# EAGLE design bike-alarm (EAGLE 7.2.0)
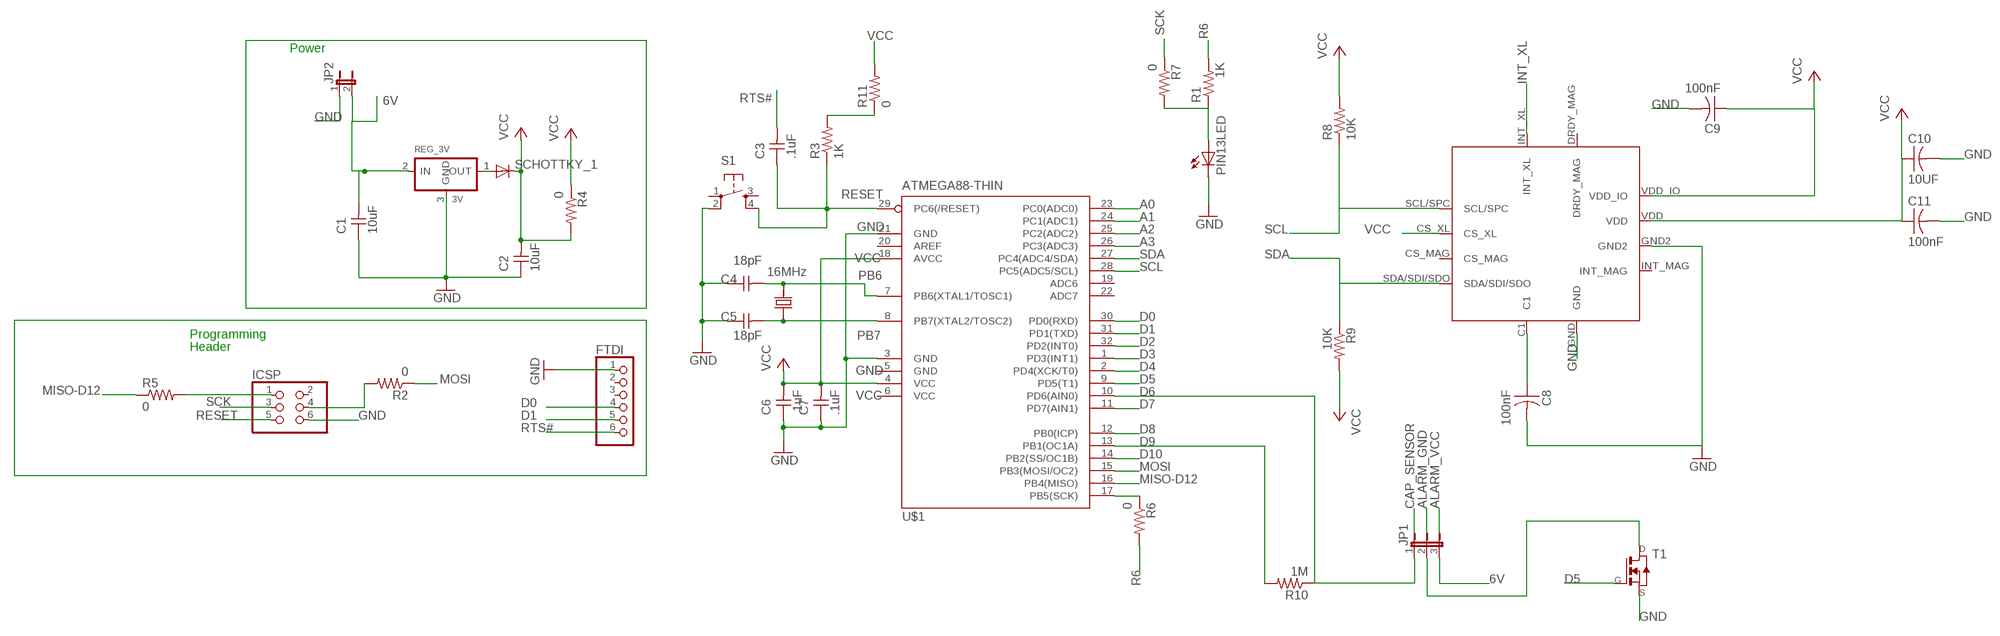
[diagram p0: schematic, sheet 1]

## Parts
C1  10uF  UNPOLARIZED_CAPACITOR1206  [1206]
C2  10uF  UNPOLARIZED_CAPACITOR1206  [1206]
C3  .1uF  UNPOLARIZED_CAPACITOR1206  [1206]
C4  18pF  UNPOLARIZED_CAPACITOR1206  [1206]
C5  18pF  UNPOLARIZED_CAPACITOR1206  [1206]
C6  .1uF  UNPOLARIZED_CAPACITOR1206  [1206]
C7  .1uF  UNPOLARIZED_CAPACITOR1206  [1206]
C8  100nF  CAP-US1206FAB  [C1206FAB]
C9  100nF  CAP-US1206FAB  [C1206FAB]
C10  10UF  CAP-US1206FAB  [C1206FAB]
C11  100nF  CAP-US1206FAB  [C1206FAB]
FTDI  PINHD-1X6  [1X06]
ICSP  PINHD-2X3-SMD  [2X03SMD]
JP1  JP2E  [JP2]
JP2  JP1E  [JP1]
PIN13LED  LED1206  [1206]
Q2  16MHz  CRYSTALCS10  [CS10]
R1  1K  RESISTOR1206  [1206]
R2  0  RES-US1206FAB  [R1206FAB]
R3  1K  RESISTOR1206  [1206]
R4  0  RES-US1206FAB  [R1206FAB]
R5  0  RES-US1206FAB  [R1206FAB]
R6  0  RES-US1206FAB  [R1206FAB]
R7  0  RES-US1206FAB  [R1206FAB]
R8  10K  RES-US1206FAB  [R1206FAB]
R9  10K  RES-US1206FAB  [R1206FAB]
R10  1M  RES-US1206FAB  [R1206FAB]
R11  0  RES-US1206FAB  [R1206FAB]
REG_3V  3V  REGULATORSOT23  [SOT23]
S1  6MM_SWITCH6MM_SWITCH  [6MM_SWITCH]
SCHOTTKY_1  DIODESOD123  [SOD123]
T1  NMOSFETSOT23  [SOT-23]
U$1  ATMEGA88-THIN  [TQFP32-08THIN]
U$3  LSM303C  [LSM303C]

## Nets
6V: C1.2 JP1.3 JP2.2 REG_3V.2(IN)
A: JP1.2 T1.1(D)
A0: U$1.23(PC0(ADC0))
A1: U$1.24(PC1(ADC1))
A2: U$1.25(PC2(ADC2))
A3: U$1.26(PC3(ADC3))
D0: FTDI.4 U$1.30(PD0(RXD))
D1: FTDI.5 U$1.31(PD1(TXD))
D2: U$1.32(PD2(INT0))
D3: U$1.1(PD3(INT1))
D4: U$1.2(PD4(XCK/T0))
D5: T1.3(G) U$1.9(PD5(T1))
D6: JP1.1 R10.1 U$1.10(PD6(AIN0))
D7: U$1.11(PD7(AIN1))
D8: U$1.12(PB0(ICP))
D9: R10.2 U$1.13(PB1(OC1A))
D10: U$1.14(PB2(SS/OC1B))
GND [power]: C1.1 C2.1 C4.1 C5.1 C6.1 C7.1 C8.2 C9.2 C10.2 C11.2 FTDI.1 ICSP.6 JP2.1 PIN13LED.2(C) REG_3V.3(GND) S1.2(P1) T1.2(S) U$1.3(GND) U$1.21(GND) U$3.GND U$3.GND2
INT_XL: U$3.INT_XL
MISO-D12: R5.1 U$1.16(PB4(MISO))
MOSI: R2.1 U$1.15(PB3(MOSI/OC2))
N$1 [power]: REG_3V.1(OUT) SCHOTTKY_1.ANODE(A)
N$4: PIN13LED.1(A) R1.1 R7.2
N$6: C8.1 U$3.C1
N$8: ICSP.4 R2.2
N$21: ICSP.1 R5.2
PB6: C4.2 Q2.P$2 U$1.7(PB6(XTAL1/TOSC1))
PB7: C5.2 Q2.P$1 U$1.8(PB7(XTAL2/TOSC2))
R6: R1.2 R6.2
RESET: C3.1 ICSP.5 R3.1 S1.4(S1) U$1.29(PC6(/RESET))
RTS#: C3.2 FTDI.6
SCK: ICSP.3 R7.1
SCK-D13: R6.1 U$1.17(PB5(SCK))
SCL: R8.1 U$1.28(PC5(ADC5/SCL)) U$3.SCL/SPC
SDA: R9.1 U$1.27(PC4(ADC4/SDA)) U$3.SDA/SDI/SDO
VCC [power]: C2.2 C6.2 C7.2 C9.1 C10.1 C11.1 R3.2 R4.1 R4.2 R8.2 R9.2 R11.1 R11.2 SCHOTTKY_1.CATHODE(C) U$1.4(VCC) U$1.18(AVCC) U$3.CS_XL U$3.VDD U$3.VDD_IO
Unconnected: FTDI.2 FTDI.3 ICSP.2 S1.1(P) S1.3(S) U$1.19(ADC6) U$1.20(AREF) U$1.22(ADC7) U$3.CS_MAG U$3.DRDY_MAG U$3.INT_MAG

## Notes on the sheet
- Power
- Programming
- Header

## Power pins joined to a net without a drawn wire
GND: U$1.5(GND)
VCC: U$1.6(VCC)

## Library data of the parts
C1-C7 = ng:UNPOLARIZED_CAPACITOR: unpolarized_capacitor
C8-C11 = fab:CAP-US
FTDI = pinhead:PINHD-1X6: PIN HEADER
ICSP = fab:PINHD-2X3-SMD: PIN HEADER
JP1 = jumper:JP2E: JUMPER
JP2 = jumper:JP1E: JUMPER
PIN13LED = ng:LED
Q2 = ng:CRYSTAL: CRYSTAL
R1 R3 = ng:RESISTOR
R2 R4-R11 = fab:RES-US: Resistor (US Symbol)
REG_3V = ng:REGULATOR
S1 = ng:6MM_SWITCH: OMRON SWITCH
SCHOTTKY_1 = 01_ng:DIODE: DIODE
T1 = fab:NMOSFET: MOS FET
U$1 = fab:ATMEGA88-THIN
U$3 = LSM303C-accelerometer:LSM303C: Ultra-Compact High-Performance e-compass 3D Accelerometer and 3D Magnetometer Module datasheet: http://www.st.com/st-web-ui/static/active/en/resource/technical/document/datasheet/DM00089896.pdf

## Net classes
0 default: width 0.635 mm, clearance 0.406 mm
1 power: width 0.635 mm, clearance 0.406 mm

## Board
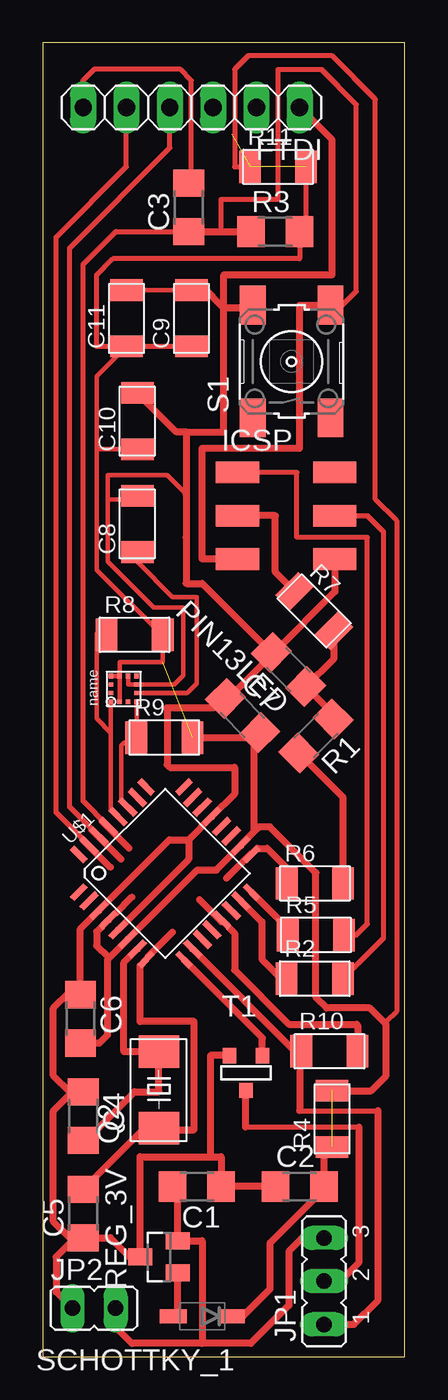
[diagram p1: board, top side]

Size 21.26 x 77.14 mm. Coordinates in mm from the lower left corner, seen from the top.
Outline: 0,0 21.26,0 21.26,77.14 0,77.14 0,0
Copper layers (1*16): Top 0.035mm / dielectric 1.5mm / Bottom 0.035mm
Design rules "default *": minimum track width 10mil, minimum drill 24mil, track to track 0.25mm, track to pad 0.25mm, pad to pad 0.25mm, via to via 0.25mm, smd to smd 0.25mm, copper to edge 40mil, drill to drill 8mil, minimum pad ring 10mil, minimum via ring 8mil, stop-mask expansion 4mil, vias tented up to drill 0mil, thermal gap 10mil

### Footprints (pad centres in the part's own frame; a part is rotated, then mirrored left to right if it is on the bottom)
1206 = smd 1.6 x 1.803: 1 -1.422,0; 2 1.422,0
C1206FAB = smd 1.27 x 1.905: 1 -1.651,0; 2 1.651,0
1X06 = drill 1.016 long: 1 -6.35,0; 2 -3.81,0; 3 -1.27,0; 4 1.27,0; 5 3.81,0; 6 6.35,0
2X03SMD = smd 2.54 x 1.27: 1 -2.857,2.54; 2 2.857,2.54; 3 -2.857,0; 4 2.857,0; 5 -2.857,-2.54; 6 2.857,-2.54
JP2 = drill 0.914 long: 1 -2.54,0; 2 0,0; 3 2.54,0
JP1 = drill 0.914 long: 1 0,-1.27; 2 0,1.27
CS10 = smd 1.905 x 2.388: P$1 -2.286,0; P$2 2.21,0
R1206FAB = smd 1.27 x 1.905: 1 -1.651,0; 2 1.651,0
SOT23 = smd 1 x 1.4: 1 -0.95,-1.1; 2 0.95,-1.1; 3 0,1.1
6MM_SWITCH = smd 2.286 x 1.524: 1 -3.302,2.286; 2 3.302,2.286; 3 -3.302,-2.286; 4 3.302,-2.286
SOD123 = smd 1.6 x 0.8: ANODE 1.7,0; CATHODE -1.7,0
SOT-23 = smd 0.787 x 0.889: 1 0.025,-1.016; 2 -0.94,1.016; 3 0.991,1.016
TQFP32-08THIN = smd 1.118 x 0.356: 1 -4.369,2.8; 8 -4.369,-2.8; 17 4.369,-2.8; 24 4.369,2.8 | smd 1.27 x 0.356: 2 -4.293,2; 3 -4.293,1.2; 4 -4.293,0.4; 5 -4.293,-0.4; 6 -4.293,-1.2; 7 -4.293,-2; 18 4.293,-2; 19 4.293,-1.2; 20 4.293,-0.4; 21 4.293,0.4; 22 4.293,1.2; 23 4.293,2 | smd 0.356 x 1.118: 9 -2.8,-4.369; 16 2.8,-4.369; 25 2.8,4.369; 32 -2.8,4.369 | smd 0.356 x 1.27: 10 -2,-4.293; 14 1.2,-4.293; 15 2,-4.293; 26 2,4.293; 27 1.2,4.293; 31 -2,4.293 | smd 0.35 x 1.27: 11 -1.2,-4.293; 12 -0.4,-4.293; 13 0.4,-4.293; 28 0.4,4.293; 29 -0.4,4.293; 30 -1.2,4.293
LSM303C = smd 0.25 x 0.275: C1 -0.25,-0.75; DRDY_MAG 0.25,0.75; GND 0.25,-0.75; INT_XL -0.25,0.75 | smd 0.275 x 0.25: CS_MAG -0.75,-0.25; CS_XL -0.75,0.25; GND2 0.75,-0.25; INT_MAG 0.75,-0.75; SCL/SPC -0.75,0.75; SDA/SDI/SDO -0.75,-0.75; VDD 0.75,0.25; VDD_IO 0.75,0.75

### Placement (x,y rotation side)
C1  9.05,10 180 top
C2  15.08,10 0 top
C3  8.57,67.47 90 top
C4  2.38,14.13 270 top
C5  2.38,8.41 90 top
C6  2.22,19.84 270 top
C7  11.73,37.64 315 top
C8  5.56,48.9 90 top
C9  8.73,60.96 90 top
C10  5.56,54.93 90 top
C11  4.92,60.96 90 top
FTDI  8.73,73.34 180 top
ICSP  14.29,49.37 0 top
JP1  16.51,4.45 90 top
JP2  3.02,2.86 270 top
PIN13LED  14.43,40.34 135 top
Q2  6.83,15.72 90 top
R1  16.03,36.45 225 top
R2  15.97,22.2 0 top
R3  13.65,66.04 0 top
R4  16.99,13.97 90 top
R5  16.03,24.77 0 top
R6  15.98,27.79 0 top
R7  15.93,43.79 315 top
R8  5.4,42.39 0 top
R9  7.14,36.35 0 top
R10  16.83,17.94 0 top
R11  13.81,69.85 0 top
REG_3V  6.83,5.87 90 top
S1  14.61,58.42 90 top
SCHOTTKY_1  9.37,2.38 180 top
T1  11.91,16.67 0 top
U$1  7.18,28.39 45 top
U$3  4.76,39.21 90 top

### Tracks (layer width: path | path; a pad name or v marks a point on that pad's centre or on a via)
6V
  Top 0.406: JP1.3 15.24,6.99 14.45,6.19 14.45,3.02 12.22,0.79 9.37,0.79 | 9.37,0.79 5.24,0.79 4.29,1.75 JP2.2 | C1.2 7.93,10 REG_3V.2 9.37,6.82 9.37,0.79
A
  Top 0.305: 11.91,13.49 18.41,13.49 18.57,13.34
  Top 0.406: JP1.2 17.46,4.45 18.57,5.56 18.57,13.34 18.57,13.49 | 11.91,13.49 11.91,15.65 T1.1
D0
  Top 0.305: U$1.30 1.59,32.29 1.59,65.09 7.46,70.96 FTDI.4
D1
  Top 0.305: U$1.31 0.79,31.95 0.79,65.72 4.92,69.85 FTDI.5
D5
  Top 0.406: T1.3 12.9,18.71 U$1.9
D6
  Top 0.305: 15.08,14.45 19.68,14.45
  Top 0.406: JP1.1 18.26,1.91 19.68,3.33 19.68,14.45 | 15.08,14.45 15.08,17.84 R10.1 14.8,17.94 U$1.10
D9
  Top 0.406: U$1.13 11.27,24.87 11.27,22.7 14.45,19.53 18.41,19.53 18.48,19.46 R10.2
GND
  Top 0.254: U$3.GND2 5.01,39.46 U$3.GND 7.71,39.46 8.26,40.01 8.26,43.97 6.51,43.97 3.81,46.67 3.81,50.32 | 3.81,50.32 3.81,51.75 7.3,51.75 8.41,50.64 | C11.2 C9.2 8.95,62.83 | C8.2 5.33,50.32 3.81,50.32
  Top 0.305: 8.41,48.26 8.41,48.1
  Top 0.406: 1.91,6.99 0.79,5.87 0.79,3.81 JP2.1 | C2.1 C1.1 10.48,11.75 9.84,11.75 | 1.91,6.99 C5.1 3.97,6.99 5.09,5.87 REG_3V.3 5.73,11.75 9.84,11.75 | 1.91,6.99 1.58,6.99 0.64,7.94 0.64,14.45 1.75,15.56 C4.1 1.59,15.55 0.64,16.51 0.64,20.48 1.59,21.43 2.22,21.43 | 2.22,21.43 C6.1 1.59,21.27 | T1.2 9.84,17.68 9.84,11.75 | 2.22,21.43 2.22,25.12 U$1.3 7.44,30.34 8.57,30.34 | U$1.5 8.57,29.21 8.57,30.34 | 8.57,30.34 U$1.21 11.27,33.04 11.27,34.61 7.46,34.61 7.3,34.77 7.3,38.1 10.02,38.1 C7.1 10.88,38.65 13.58,41.35 | ICSP.6 17.14,44.91 13.58,41.35 | 13.58,41.35 PIN13LED.2 9.37,45.4 8.41,45.4 8.41,48.1 8.41,50.64 8.41,54.29 | 8.41,54.29 10.64,54.29 10.64,61.56 | 8.41,54.29 7.84,54.29 C10.2 | 8.95,62.83 9.37,62.83 10.64,61.56 | 10.64,61.56 10.64,63.5 16.99,63.5 16.99,71.44 FTDI.1 | S1.2 12.32,61.56 10.64,61.56
MISO-D12
  Top 0.406: U$1.16 14.38,25.15 R5.1
MOSI
  Top 0.406: U$1.15 12.86,25.54 12.86,23.34 14,22.2 R2.1
N$1
  Top 0.406: SCHOTTKY_1.ANODE 7.92,2.38 REG_3V.1
N$4
  Top 0.406: R1.1 17.04,37.73 PIN13LED.1 17.1,41 R7.2
N$6
  Top 0.254: C8.1 5.56,46.67 7.62,44.61 9.05,44.61 9.05,39.53 8.48,38.96 U$3.C1
N$8
  Top 0.305: R2.2 20,24.58 20,48.42 19.05,49.37 ICSP.4
N$12  (2 unrouted)
  Top 0.305: 20.16,19.68 20.8,20.32 20.8,49.05 19.53,50.32 19.53,73.82 16.99,76.36 12.06,76.36 11.27,75.56 11.27,69.85 12.22,69.85
N$14
  Top 0.406: 3.49,31.43 5.08,29.84
N$15
  Top 0.406: 2.86,30.96 4.6,29.21
N$16
  Top 0.406: 2.38,30.32 3.97,28.73
N$17
  Top 0.406: 10.48,25.56 9.21,26.83
N$18
  Top 0.406: 6.19,23.5 7.62,24.92
N$19
  Top 0.406: 4.29,26.04 5.24,26.99
N$20
  Top 0.406: 12.22,29.53 10.79,28.1
N$21
  Top 0.305: R5.2 18.41,24.77 19.05,25.4 19.05,48.1 14.92,48.1 14.92,51.91 ICSP.1
PB6
  Top 0.406: C4.2 2.55,12.71 5.4,15.56 6.83,15.56 Q2.P$2 4.76,17.93 4.76,23.14 U$1.7
PB7
  Top 0.406: C5.2 5.87,13.34 6.73,13.34 Q2.P$1 6.83,13.34 8.89,13.34 8.89,19.68 5.71,19.68 5.71,22.96 U$1.8
R6
  Top 0.406: R6.2 17.63,32.84 R1.2
RESET
  Top 0.305: 10.48,66.05 10.48,67.94 13.81,67.94 13.81,75.56 16.35,75.56 18.41,73.5 18.41,62.55 17.59,61.72 S1.4 | U$1.29 2.38,32.62 2.38,64.14 4.29,66.05 C3.1
  Top 0.406: ICSP.5 9.37,46.83 9.37,53.34 15.08,53.34 15.08,61.72 S1.4 | C3.1 10.48,66.05 10.49,66.05 R3.1
RTS#
  Top 0.305: FTDI.6 2.38,74.93 3.02,75.56 8.1,75.56 8.73,74.93 8.73,68.89 C3.2
SCK
  Top 0.406: R7.1 13.65,46.06 13.65,49.37 ICSP.3
SCK-D13
  Top 0.406: U$1.17 12.6,29.84 13.18,29.84 14.32,28.7 R6.1
SCL
  Top 0.254: U$1.28 4.01,32.12 4.01,36.63 | 4.01,36.63 U$3.SCL/SPC | R8.1 3.17,42.45 3.17,37.47 4.01,36.63
SDA
  Top 0.254: U$3.SDA/SDI/SDO 5.51,36.06 R9.1 4.76,36.04 4.6,35.88 4.6,32.66 U$1.27
VCC  (3 unrouted)
  Top 0.254: U$3.VDD_IO U$3.VDD | U$3.VDD 4.51,40.8 7.05,40.8 R8.2 | R8.2 7.05,42.55 | 3.17,53.28 3.17,46.2 6.99,42.39 R8.2 | 3.17,53.28 C10.1 | 3.17,53.28 3.17,57.56 C11.1 C9.1 | U$3.VDD U$3.CS_XL
  Top 0.305: C9.1 3.17,59.31 3.17,63.5 4.13,64.45 15.07,64.45 R3.2 | 15.46,66.43 R11.2
  Top 0.406: C6.2 2.39,18.41 3.33,18.41 3.81,18.89 3.81,23.32 | 3.81,23.32 U$1.6 9.06,28.57 10.2,28.57 U$1.18 11.63,30.05 12.38,30.8 | U$1.4 3.17,24.95 3.17,24.13 3.81,23.5 3.81,23.32 | C7.2 12.38,36.29 | 12.38,36.29 12.38,30.8 | R9.2 11.97,36.35 12.38,36.29 | 12.38,30.8 12.7,31.11 13.34,31.11 16.03,28.42 16.03,21.11 16.67,20.48 19.21,20.48 20.16,19.53 20.16,16.51 19.27,15.62 R4.2 | SCHOTTKY_1.CATHODE 11.75,2.38 13.34,3.97 13.34,6.67 16.5,9.84 C2.2 16.5,11.84 R4.1 | R3.2 15.46,66.43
